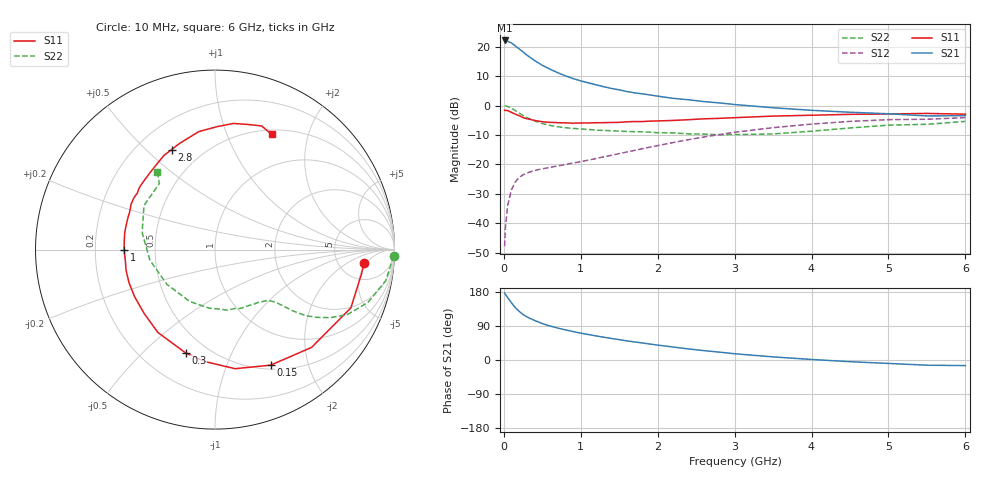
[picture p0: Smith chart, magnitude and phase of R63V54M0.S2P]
! SIEMENS Small Signal Semiconductors
! BFR193
! Si NPN RF Bipolar Junction Transistor in SOT23
! VCE = 3.5 V  IC = 4 mA
! Common Emitter S-Parameters:  May  1996
# GHz  S  MA  R  50
!  f  S11  S21  S12  S22
! GHz  MAG  ANG  MAG  ANG  MAG  ANG  MAG  ANG
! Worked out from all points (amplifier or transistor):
!   36 points, 10 MHz to 6 GHz, reference 50 ohm
!   highest |S21| = 22.1 dB at 10 MHz (marker M1)
!   |S21| within 3 dB of that: start of sweep to 206 MHz
!   unconditionally stable (mu >= 1): 965 MHz to 2.036 GHz
!   at 250 MHz: K = 0.37, MSG = 20.9 dB, |S12| = -23.5 dB
!   at 1.4 GHz: K = 1.07, MAG = 9.7 dB, |S12| = -16.9 dB
!   at 6 GHz: K = 0.98, MSG = 0.3 dB, |S12| = -4.1 dB
!   S11 on the Smith chart (normalised r, x): 10 MHz: 8.97, -4.28; 150 MHz: 0.55, -1.45; 300 MHz: 0.38, -0.68; 1 GHz: 0.33, -0.00; 2.8 GHz: 0.34, +0.60; 6 GHz: 0.56, +1.46
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0.01  0.8338 -5.0  12.77 177.1  0.0041 88.6  0.9954 -2.0
0.02  0.8276 -9.3  12.62 173.6  0.0084 82.7  0.9865 -4.2
0.05  0.8237 -23.2  12.35 164.6  0.0202 77.9  0.9671 -10.3
0.1  0.7657 -45.4  11.59 150.5  0.0374 68.3  0.9011 -19.1
0.15  0.7144 -64.3  10.26 138.0  0.0509 59.8  0.822 -26.1
0.2  0.673 -80.4  9.173 128.3  0.0604 54.2  0.7473 -30.5
0.25  0.6265 -95.1  8.138 120.0  0.0666 49.6  0.6765 -33.9
0.3  0.5984 -105.9  7.202 113.8  0.0716 47.3  0.6233 -36.1
0.4  0.5605 -124.7  5.818 104.3  0.0793 44.2  0.5491 -38.3
0.5  0.5312 -138.1  4.833 96.1  0.0844 43.8  0.4966 -39.5
0.6  0.5191 -149.7  4.153 89.7  0.0894 44.5  0.4605 -40.5
0.7  0.5133 -159.0  3.622 84.3  0.0943 46.0  0.4378 -41.6
0.8  0.5088 -166.8  3.2 79.5  0.0999 47.2  0.4208 -42.8
1  0.5064 -179.9  2.629 70.9  0.1115 50.8  0.401 -45.4
1.1  0.508 174.2  2.43 67.2  0.1187 52.6  0.3928 -47.5
1.6  0.5314 151.7  1.732 50.4  0.1631 58.2  0.3636 -59.2
2.2  0.5599 130.7  1.329 34.3  0.2354 58.5  0.344 -78.5
2.8  0.6073 113.5  1.111 20.8  0.3222 52.8  0.3197 -105.3
3.5  0.6636 97.8  0.919 8.2  0.4221 42.0  0.3304 -143.9
4.5  0.7103 81.7  0.771 -4.4  0.5392 24.3  0.417 166.8
5.5  0.7363 69.3  0.668 -13.7  0.5868 6.5  0.4813 130.1
6  0.7152 63.8  0.674 -14.8  0.6238 1.5  0.5389 126.6
